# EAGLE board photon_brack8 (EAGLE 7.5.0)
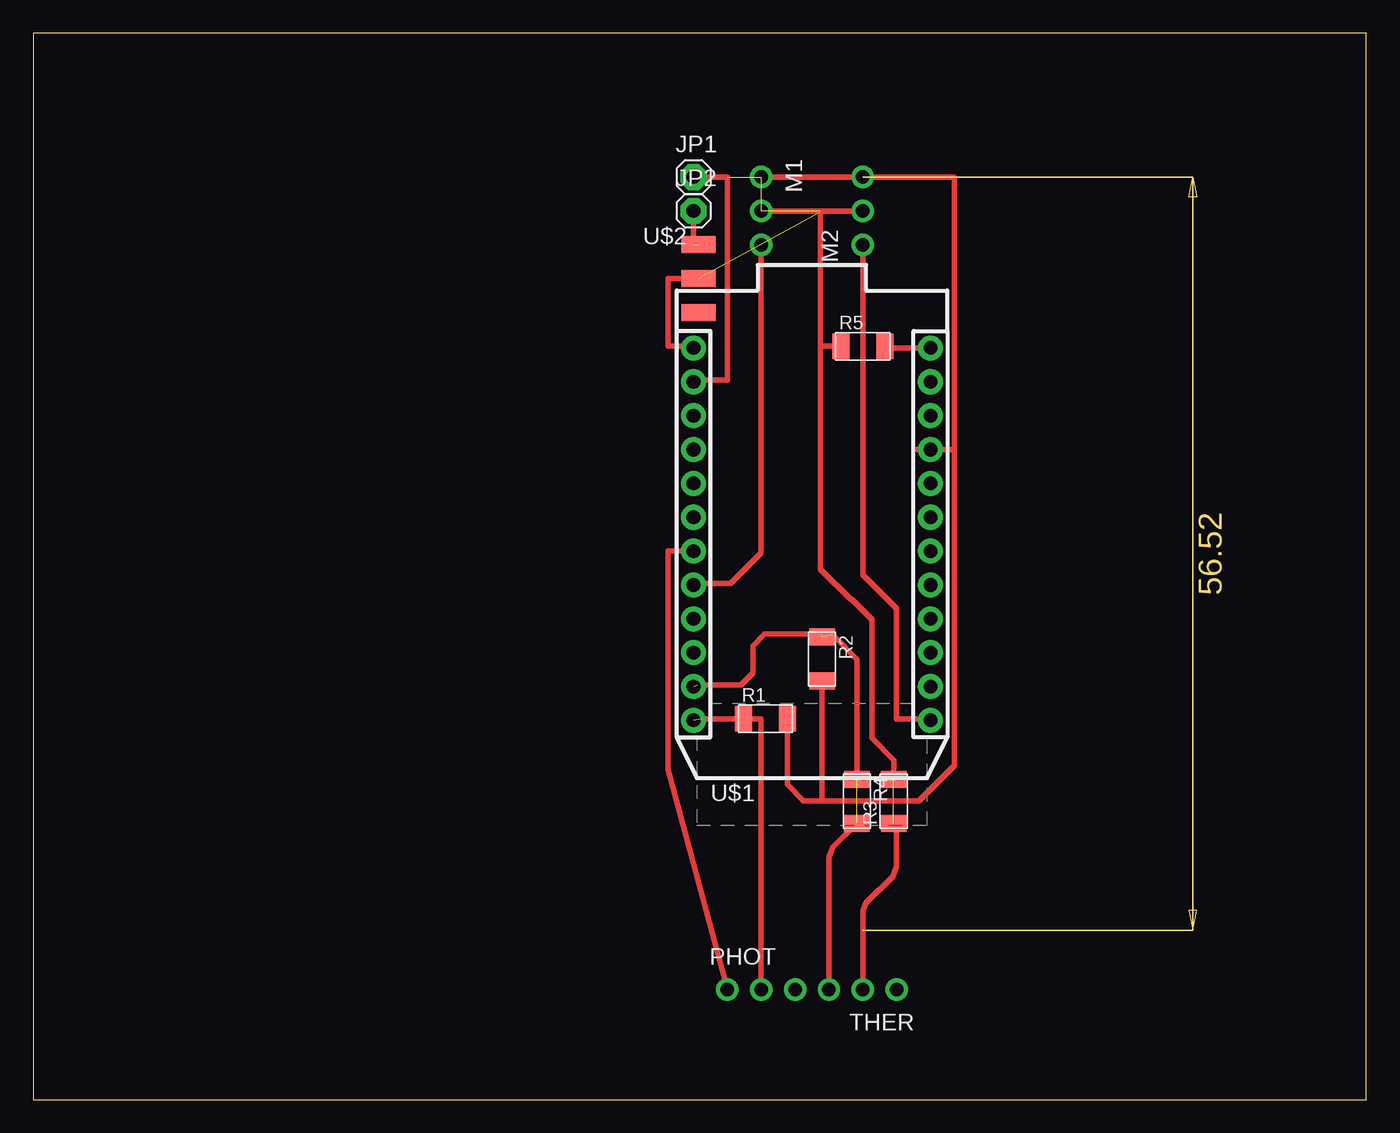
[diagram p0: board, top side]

Size 100 x 80 mm. Coordinates in mm from the lower left corner, seen from the top.
Outline: 0,0 100,0 100,80 0,80 0,0
Copper layers (1*16): Top 0.035mm / dielectric 1.5mm / Bottom 0.035mm
Design rules "default": minimum track width 10mil, minimum drill 24mil, track to track 8mil, track to pad 8mil, pad to pad 8mil, via to via 8mil, smd to smd 8mil, copper to edge 40mil, drill to drill 8mil, minimum pad ring 10mil, minimum via ring 8mil, stop-mask expansion 4mil, vias tented up to drill 0mil, thermal gap 10mil
Net classes: 2 RF: width 0.381 mm, clearance 0.381 mm

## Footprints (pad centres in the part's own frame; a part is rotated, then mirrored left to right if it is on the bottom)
1X01 = drill 1.016 pad 1.93 octagon: 1 0,0
1X03-CLEANBIG = drill 1.016 pad 1.676: 1 -2.54,0; 2 0,0; 3 2.54,0
R1206FAB = smd 1.27 x 1.905: 1 -1.651,0; 2 1.651,0
PHOTON = drill 1.016 pad 1.88: 1 1.27,32.258; 2 1.27,29.718; 3 1.27,27.178; 4 1.27,24.638; 5 1.27,22.098; 6 1.27,19.558; 7 1.27,17.018; 8 1.27,14.478; 9 1.27,11.938; 10 1.27,9.398; 11 1.27,6.858; 12 1.27,4.318; 13 19.05,4.318; 14 19.05,6.858; 15 19.05,9.398; 16 19.05,11.938; 17 19.05,14.478; 18 19.05,17.018; 19 19.05,19.558; 20 19.05,22.098; 21 19.05,24.638; 22 19.05,27.178; 23 19.05,29.718; 24 19.05,32.258
SPDTSWITCH = smd 2.54 x 1.27: 1 0.38,2.54; 2 0.38,0; 3 0.38,-2.54

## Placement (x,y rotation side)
JP1  [1X01]  49.53,69.22 0 top
JP2  [1X01]  49.53,66.67 0 top
M1  [1X03-CLEANBIG]  54.61,66.67 270 top
M2  [1X03-CLEANBIG]  62.23,66.67 90 top
PHOT  [1X03-CLEANBIG]  54.61,8.26 0 top
R1  [R1206FAB]  54.93,28.57 0 top
R2  [R1206FAB]  59.18,33.05 270 top
R3  0  [R1206FAB]  64.55,22.38 90 top
R4  0  [R1206FAB]  61.79,22.38 270 top
R5  0  [R1206FAB]  62.23,56.52 0 top
THER  [1X03-CLEANBIG]  62.23,8.26 180 top
U$1  PHOTON_WITH_HEADERS  [PHOTON]  48.26,24.13 0 top
U$2  SPDTSWITCH  [SPDTSWITCH]  49.53,61.59 0 top

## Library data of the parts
JP1 JP2 M1 M2 PHOT THER = adafruit
R1-R5 U$2 = 01fab
U$1 = Spark

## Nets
3V3: R5.2 U$1.24
A0: PHOT.2 R1.1 U$1.12
A1: R2.1 R4.1 R4.2 THER.3 U$1.11
A4: M1.3 U$1.8
A5: PHOT.1 U$1.7
D0: U$1.13
GND [vcc]: JP1.1 M1.1 M2.3 R1.2 R2.2 U$1.2 U$1.21
N$1 [vcc]: M1.2 M2.2 R5.1
N$2: JP2.1 U$2.1
N$3: M2.1
N$4: U$1.3
N$5: U$1.4
N$6: U$1.5
N$7: U$1.6
N$11: U$1.10
N$15: U$1.23
N$16: U$1.22
N$20: U$1.18
N$21: U$1.17
N$22: U$1.16
N$24: U$1.14
VIN [vcc]: R3.1 R3.2 THER.2 U$1.1 U$2.2

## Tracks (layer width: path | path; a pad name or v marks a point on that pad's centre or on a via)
3V3
  Top 0.406: U$1.24 63.88,56.39 R5.2
A0  (1 unrouted)
  Top 0.406: 50.16,28.57 R1.1 54.61,28.57 PHOT.2
A1  (4 unrouted)
  Top 0.406: 49.85,31.11 53.08,31.11 53.98,32.01 53.98,34.03 54.87,34.92 59.05,34.92 | R4.1 61.78,33.02 59.98,34.86 | R4.2 60,18.95 59.69,18.2 THER.3
A4
  Top 0.406: U$1.8 49.53,38.73 52.32,38.73 54.61,41.02 M1.3
A5
  Top 0.406: U$1.7 47.62,41.15 47.62,24.77 PHOT.1
GND  (2 unrouted)
  Top 0.406: 62.23,66.67 54.61,66.67 | 66.31,48.77 U$1.21 69.09,48.77 | 62.97,69.22 M2.3 | M1.1 M2.3 | R1.2 56.58,23.64 57.8,22.42 59.18,22.42 | 59.18,22.42 66.44,22.42 69.09,25.06 69.09,48.77 | R2.2 59.18,22.42 | 69.09,48.77 69.09,69.22 M2.3 | U$1.2 49.53,53.98 52.07,53.98 52.07,67.31 52.07,68.58 52.07,69.22 JP1.1
N$1  (1 unrouted)
  Top 0.406: R5.1 59.05,56.52 59.05,66.67 M2.2
N$2  (1 unrouted)
  Top 0.406: JP2.1 49.53,64.14
N$3
  Top 0.406: 66.67,28.57 64.77,28.57 64.77,36.83 62.23,39.37 M2.1
VIN  (2 unrouted)
  Top 0.406: R3.1 64.77,20.32 64.77,17.44 64.48,16.75 62.47,14.74 62.23,14.15 THER.2 | R3.2 64.58,25.43 62.9,27.11 62.92,36.01 61.41,37.52 61.34,37.52 59.05,39.78 59.05,66.58 | U$2.2 47.62,61.59 47.62,56.52 49.53,56.52 U$1.1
